TYPE ST_MainStructure :
STRUCT
	{attribute 'ElementName' := '_id'}
    ID: T_ObjectId_MongoDB;
    {attribute 'ElementName' := 'myBool'}
    myBool: BOOL;
    {attribute 'ElementName' := 'Name'}
    Name : STRING(256);
    {attribute 'ElementName' := 'Value'}
	Value : LREAL;
	{attribute 'ElementName' := 'Value2'}
	Value2 : LINT;
	{attribute 'ElementName' := 'Child'}
	Child : ST_ChildStructure;
	{attribute 'ElementName' := 'Children'}
	Children : ARRAY[0..2] OF ST_ChildStructure;
END_STRUCT
END_TYPE
